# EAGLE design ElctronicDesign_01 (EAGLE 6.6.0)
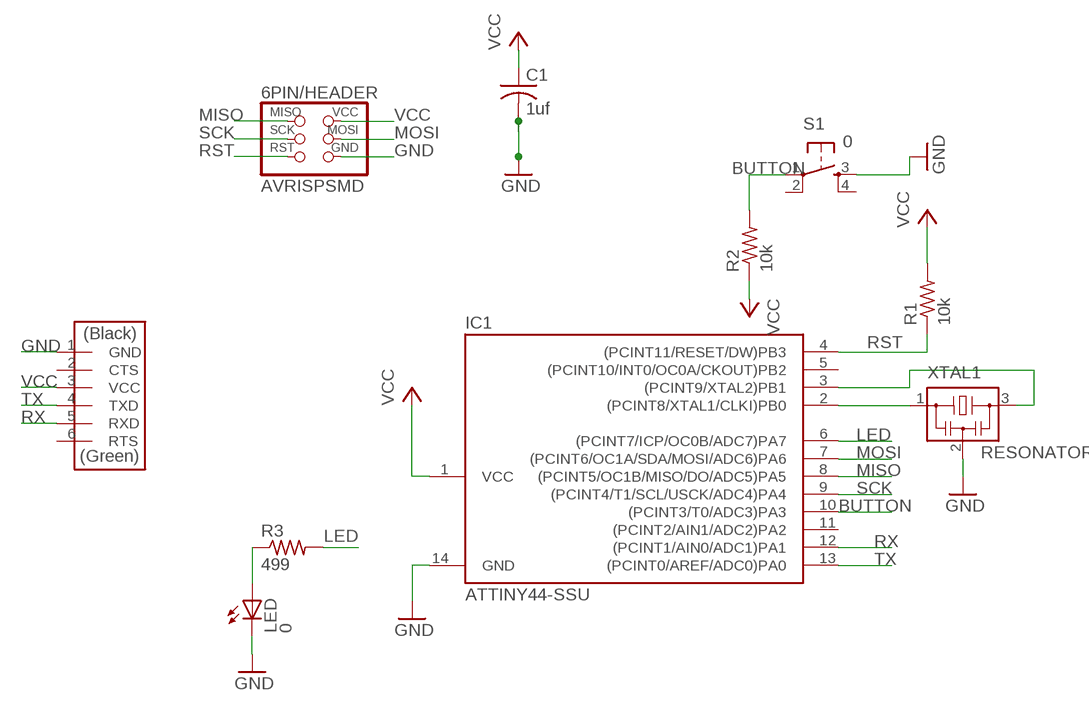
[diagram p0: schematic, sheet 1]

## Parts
6PIN/HEADER  AVRISPSMD  [2X03SMD]
C1  1uf  C-USC1206  [C1206]
IC1  ATTINY44-SSU  [SOIC14]
JP1  FTDI-SMD-HEADER  [1X06SMD]
LED  0  LED1206  [1206]
R1  10k  R-US_R1206  [R1206]
R2  10k  R-US_R1206  [R1206]
R3  499  RES-US1206FAB  [R1206FAB]
S1  0  6MM_SWITCH6MM_SWITCH  [6MM_SWITCH]
XTAL1  RESONATOR  [EFOBM]

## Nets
BUTTON: IC1.10((PCINT3/T0/ADC3)PA3) R2.2 S1.1(P)
GND: 6PIN/HEADER.6(GND) C1.2 IC1.14(GND) JP1.1(GND) LED.2(C) S1.3(S) XTAL1.2
LED: IC1.6((PCINT7/ICP/OC0B/ADC7)PA7) R3.2
MISO: 6PIN/HEADER.1(MISO) IC1.8((PCINT5/OC1B/MISO/DO/ADC5)PA5)
MOSI: 6PIN/HEADER.4(MOSI) IC1.7((PCINT6/OC1A/SDA/MOSI/ADC6)PA6)
N$1: IC1.2((PCINT8/XTAL1/CLKI)PB0) XTAL1.1
N$2: IC1.3((PCINT9/XTAL2)PB1) XTAL1.3
N$3: LED.1(A) R3.1
RST: 6PIN/HEADER.5(RST) IC1.4((PCINT11/RESET/DW)PB3) R1.1
RX: IC1.12((PCINT1/AIN0/ADC1)PA1) JP1.5(RXD)
SCK: 6PIN/HEADER.3(SCK) IC1.9((PCINT4/T1/SCL/USCK/ADC4)PA4)
TX: IC1.13((PCINT0/AREF/ADC0)PA0) JP1.4(TXD)
VCC: 6PIN/HEADER.2(VCC) C1.1 IC1.1(VCC) JP1.3(VCC) R1.2 R2.1
Unconnected: IC1.5((PCINT10/INT0/OC0A/CKOUT)PB2) IC1.11((PCINT2/AIN1/ADC2)PA2) JP1.2(CTS) JP1.6(RTS) S1.2(P1) S1.4(S1)

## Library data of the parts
6PIN/HEADER = fab:AVRISP
C1 = rcl:C-US: CAPACITOR, American symbol
IC1 = fab:ATTINY44
JP1 = fab:FTDI-SMD-HEADER
LED = ng:LED
R1 R2 = resistor:R-US_: RESISTOR, American symbol
R3 = fab:RES-US: Resistor (US Symbol)
S1 = fab:6MM_SWITCH: OMRON SWITCH
XTAL1 = fab:RESONATOR

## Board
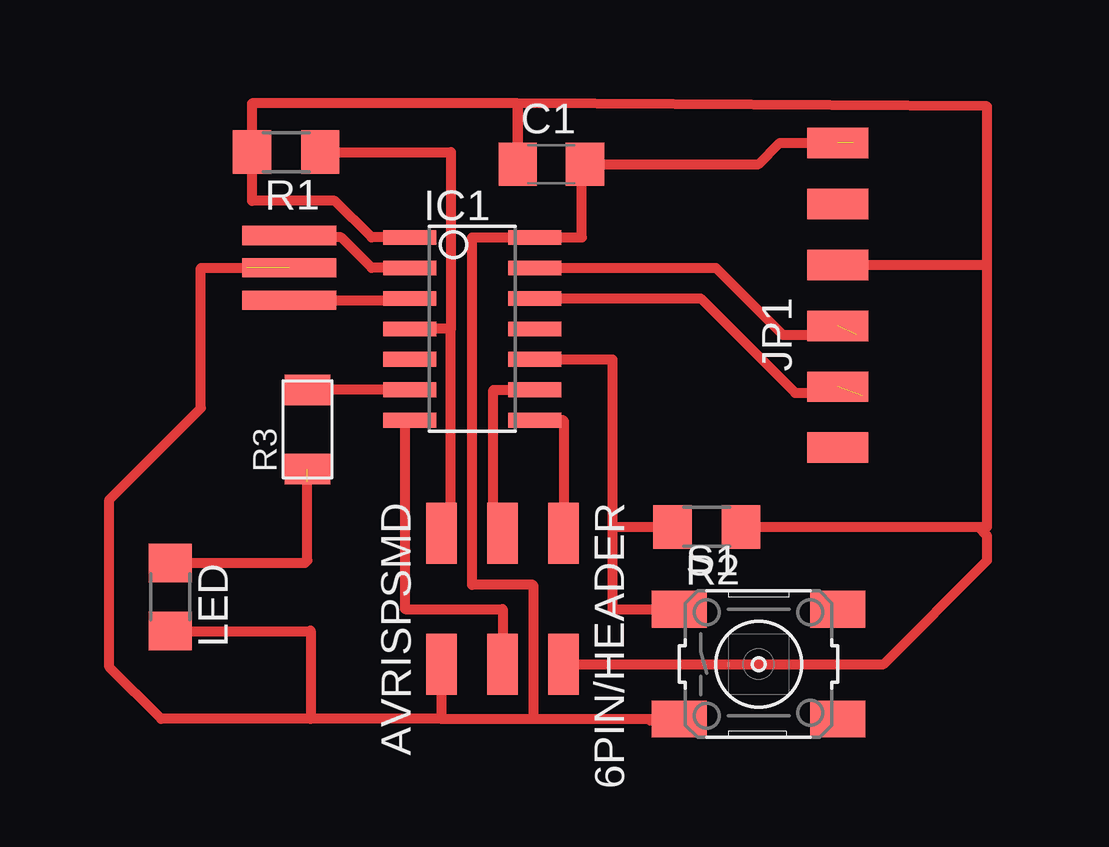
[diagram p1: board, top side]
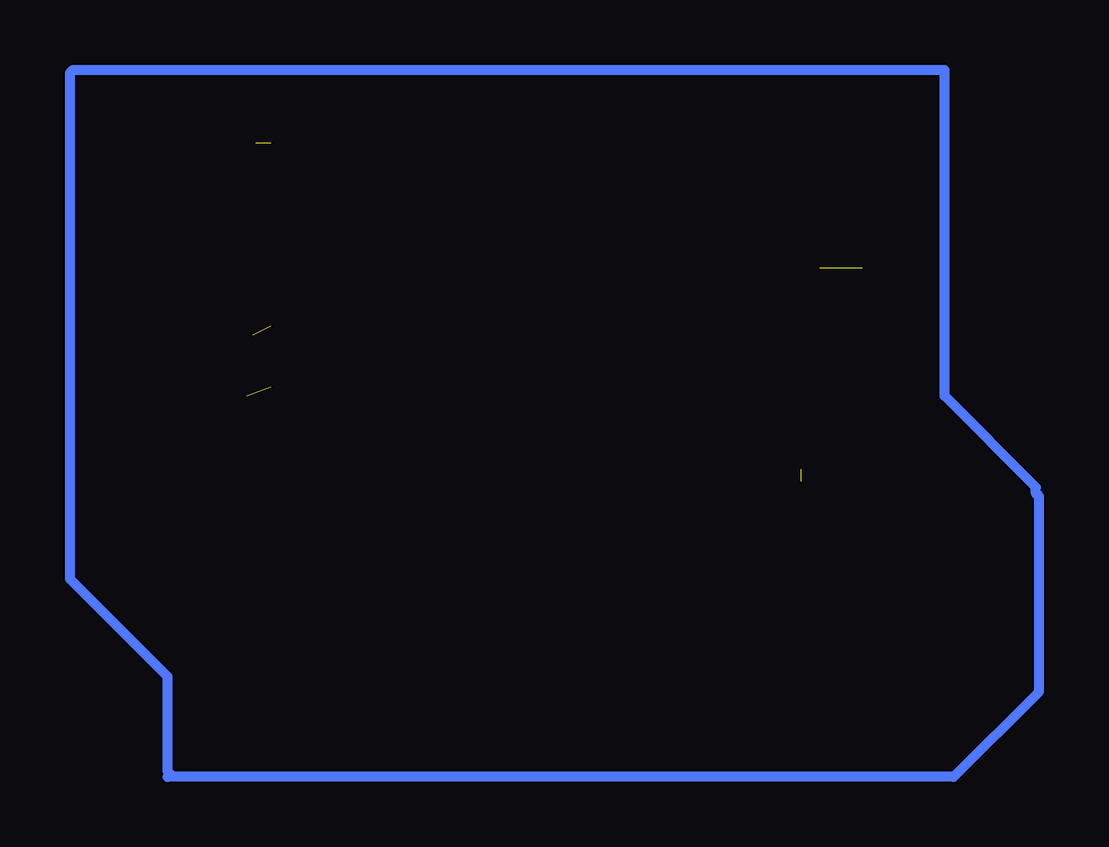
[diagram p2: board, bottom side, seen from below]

No outline drawn. Coordinates in mm, seen from the top.
Copper layers 1: Top 0.035mm
Design rules "ERP-1sided-10mil-16mill": minimum track width 10mil, minimum drill 24mil, track to track 16mil, track to pad 16mil, pad to pad 16mil, via to via 16mil, smd to smd 0mil, copper to edge 16mil, drill to drill 36mil, minimum pad ring 10mil, minimum via ring 8mil, stop-mask expansion 4mil, vias tented up to drill 0mil, thermal gap 10mil

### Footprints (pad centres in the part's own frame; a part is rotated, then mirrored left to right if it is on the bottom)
2X03SMD = smd 2.54 x 1.27: 1 -2.54,2.54; 2 2.92,2.54; 3 -2.54,0; 4 2.92,0; 5 -2.54,-2.54; 6 2.92,-2.54
C1206 = smd 1.6 x 1.8: 1 -1.4,0; 2 1.4,0
SOIC14 = smd 0.61 x 2.21: 1 -3.81,-2.603; 2 -2.54,-2.603; 3 -1.27,-2.603; 4 0,-2.603; 5 1.27,-2.603; 6 2.54,-2.603; 7 3.81,-2.603; 8 3.81,2.603; 9 2.54,2.603; 10 1.27,2.603; 11 0,2.603; 12 -1.27,2.603; 13 -2.54,2.603; 14 -3.81,2.603
1X06SMD = smd 2.54 x 1.27: 1 0,6.35; 2 0,3.81; 3 0,1.27; 4 0,-1.27; 5 0,-3.81; 6 0,-6.35
1206 = smd 1.6 x 1.803: 1 -1.422,0; 2 1.422,0
R1206 = smd 1.6 x 1.803: 1 -1.422,0; 2 1.422,0
R1206FAB = smd 1.27 x 1.905: 1 -1.651,0; 2 1.651,0
6MM_SWITCH = smd 2.286 x 1.524: 1 -3.302,2.286; 2 3.302,2.286; 3 -3.302,-2.286; 4 3.302,-2.286
EFOBM = smd 0.8 x 3.9: 1 -1.35,0; 2 0,0; 3 1.35,0

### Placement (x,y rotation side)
6PIN/HEADER  14.22,7.87 270 top
C1  16.26,25.78 0 top
IC1  12.95,18.92 270 top
JP1  28.19,20.32 0 top
LED  0.38,7.75 270 top
R1  5.21,26.29 180 top
R2  22.73,10.67 180 top
R3  6.1,14.73 90 top
S1  24.89,4.95 0 top
XTAL1  5.33,21.46 270 top

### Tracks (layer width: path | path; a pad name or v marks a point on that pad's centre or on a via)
BUTTON
  Top 0.406: IC1.10 18.8,17.65 18.8,10.67 | 18.8,10.67 18.8,7.24 S1.1 | 18.8,10.67 R2.2
GND  (2 unrouted)
  Top 0.254: S1.3 21.59,2.54 20.32,2.54 20.32,2.67
  Top 0.406: 15.49,2.67 15.49,8.26 12.95,8.26 12.95,22.73 IC1.14 17.53,22.73 17.53,25.78 C1.2 | 11.68,2.67 15.49,2.67 | C1.2 17.66,25.65 | 11.68,5.84 6PIN/HEADER.6 11.68,2.67 | 15.49,2.67 20.32,2.67 20.45,2.67 | C1.2 24.89,25.78 25.78,26.67 28.83,26.67 29.08,26.42 | 11.68,2.67 6.22,2.67 | 6.22,2.67 0,2.67 -2.16,4.83 -2.16,11.81 1.65,15.62 1.65,21.46 3.56,21.46 | LED.2 6.2,6.33 6.22,6.35 6.22,2.67
LED
  Top 0.406: IC1.6 R3.2
MISO
  Top 0.406: IC1.8 16.76,15.11 6PIN/HEADER.1
MOSI
  Top 0.406: IC1.7 10.16,15.11 10.16,7.24 14.22,7.24 6PIN/HEADER.4
N$1
  Top 0.406: IC1.2 8.76,21.46 7.49,22.73 5.41,22.73 XTAL1.1
N$2
  Top 0.406: XTAL1.3 10.35,20.11 IC1.3
N$3  (1 unrouted)
  Top 0.406: LED.1 5.99,9.17 6.1,9.27 6.1,12.57
N$4
  Bottom 0.406: 32.51,0.25 -0.25,0.25 -3.81,3.81 -3.81,11.94 -3.68,12.06 -3.68,12.32 0.13,16.13 0.13,29.59 0.25,29.72 | 0.25,29.72 36.45,29.72 36.58,29.59 36.58,8.51 32.51,4.45 32.51,0.51 32.38,0.38 | 0.25,29.72 0.13,29.72
RST
  Top 0.406: 12.06,18.92 IC1.4 | 6PIN/HEADER.5 12.06,11.3 12.06,18.92 | R1.1 12.06,26.29 12.06,18.92
RX  (1 unrouted)
  Top 0.406: IC1.12 22.48,20.19 26.42,16.26 29.08,16.26 29.21,16.13
SCK
  Top 0.406: 6PIN/HEADER.3 13.84,11.3 13.84,16.38 IC1.9
TX  (1 unrouted)
  Top 0.406: IC1.13 23.11,21.46 25.91,18.67 28.96,18.67
VCC
  Top 0.406: 34.42,21.72 34.42,10.67 34.04,10.67 | 34.42,21.72 34.42,28.19 14.86,28.32 C1.1 14.86,28.32 3.79,28.32 R1.2 3.79,24.26 7.24,24.26 8.76,22.73 IC1.1 9.65,22.73 | 6PIN/HEADER.2 30.1,4.95 34.42,9.27 34.42,10.29 34.04,10.67 | R2.1 34.04,10.67 | JP1.3 34.29,21.59 34.42,21.72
